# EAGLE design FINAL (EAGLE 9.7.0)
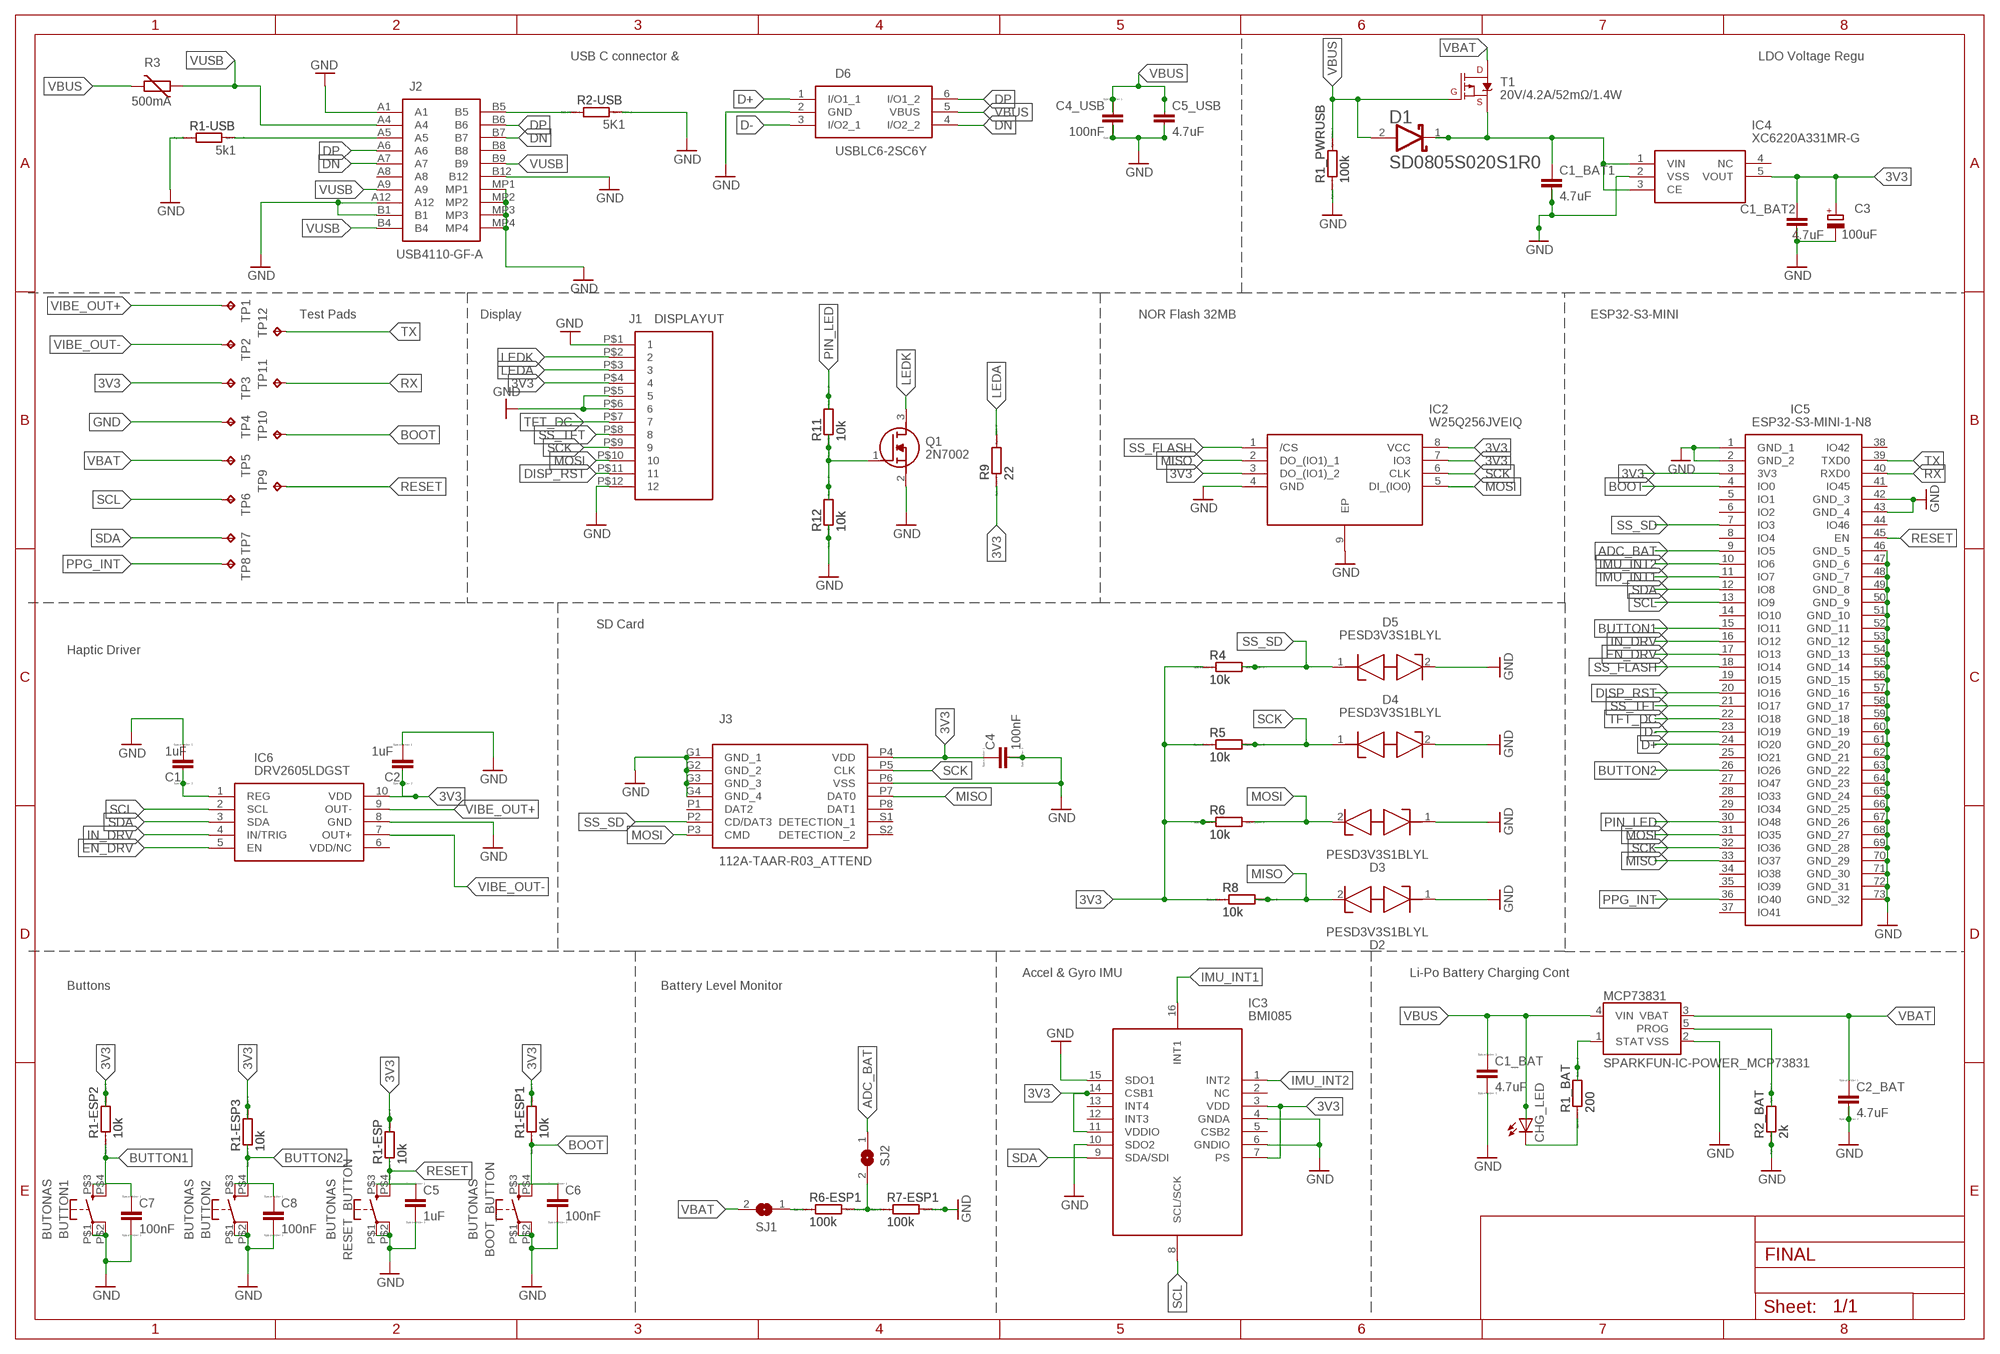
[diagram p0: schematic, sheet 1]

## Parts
BOOT_BUTTON  BUTONAS  [BUTONAS]
BUTTON1  BUTONAS  [BUTONAS]
BUTTON2  BUTONAS  [BUTONAS]
C1  1uF  EAGLE-LTSPICE_CC0402  [EAGLE-LTSPICE_C0402]
C1_BAT  4.7uF  EAGLE-LTSPICE_CC0402  [EAGLE-LTSPICE_C0402]
C1_BAT1  4.7uF  RCL_C-EUC0603  [RCL_C0603]
C1_BAT2  4.7uF  RCL_C-EUC0603  [RCL_C0603]
C2  1uF  EAGLE-LTSPICE_CC0402  [EAGLE-LTSPICE_C0402]
C2_BAT  4.7uF  EAGLE-LTSPICE_CC0402  [EAGLE-LTSPICE_C0402]
C3  100uF  CPOL-EUCT3528  [CT3528]
C4  100nF  EAGLE-LTSPICE_CC0402  [EAGLE-LTSPICE_C0402]
C4_USB  100nF  EAGLE-LTSPICE_CC0402  [EAGLE-LTSPICE_C0402]
C5  1uF  EAGLE-LTSPICE_CC0402  [EAGLE-LTSPICE_C0402]
C5_USB  4.7uF  RCL_C-EUC0603  [RCL_C0603]
C6  100nF  EAGLE-LTSPICE_CC0402  [EAGLE-LTSPICE_C0402]
C7  100nF  EAGLE-LTSPICE_CC0402  [EAGLE-LTSPICE_C0402]
C8  100nF  EAGLE-LTSPICE_CC0402  [EAGLE-LTSPICE_C0402]
CHG_LED  ADAFRUIT_LEDCHIP-LED0603  [ADAFRUIT_CHIP-LED0603]
D1  AVX---SD0805S020S1R0_AVX_SD0805S020S1R0AVX_SD0805S020S1R0_0_0  [AVX---SD0805S020S1R0_AVX_SD0805S020S1R0_0]
D2  PESD3V3S1BLYL  [PESD5V0S1BL315]
D3  PESD3V3S1BLYL  [PESD5V0S1BL315]
D4  PESD3V3S1BLYL  [PESD5V0S1BL315]
D5  PESD3V3S1BLYL  [PESD5V0S1BL315]
D6  USBLC6-2SC6Y  [SOT95P280X145-6N]
IC2  W25Q256JVEIQ  [SON127P800X600X80-9N]
IC3  BMI085  [BMI085]
IC4  XC6220A331MR-G  [SOT95P280X120-5N]
IC5  ESP32-S3-MINI-1-N8  [ESP32S3MINI1N8]
IC6  DRV2605LDGST  [SOP50P490X110-10N]
J1  DISPLAYUT  [DISPLAYUT]
J2  USB4110-GF-A  [USB4110GFA]
J3  112A-TAAR-R03_ATTEND  [112ATAARR03ATTEND]
MCP73831  SPARKFUN-IC-POWER_MCP73831  [SPARKFUN-IC-POWER_SOT23-5]
Q1  2N7002  [SOT96P240X120-3N]
R1-ESP  10k  EAGLE-LTSPICE_RR0402  [EAGLE-LTSPICE_R0402]
R1-ESP1  10k  EAGLE-LTSPICE_RR0402  [EAGLE-LTSPICE_R0402]
R1-ESP2  10k  EAGLE-LTSPICE_RR0402  [EAGLE-LTSPICE_R0402]
R1-ESP3  10k  EAGLE-LTSPICE_RR0402  [EAGLE-LTSPICE_R0402]
R1-USB  5k1  EAGLE-LTSPICE_RR0402  [EAGLE-LTSPICE_R0402]
R1_BAT  200  EAGLE-LTSPICE_RR0402  [EAGLE-LTSPICE_R0402]
R1_PWRUSB  100k  EAGLE-LTSPICE_RR0402  [EAGLE-LTSPICE_R0402]
R2-USB  5K1  EAGLE-LTSPICE_RR0402  [EAGLE-LTSPICE_R0402]
R2_BAT  2k  EAGLE-LTSPICE_RR0402  [EAGLE-LTSPICE_R0402]
R3  500mA  VARISTOR_VARISTORCN1812  [VARISTOR_CT/CN1812]
R4  10k  EAGLE-LTSPICE_RR0402  [EAGLE-LTSPICE_R0402]
R5  10k  EAGLE-LTSPICE_RR0402  [EAGLE-LTSPICE_R0402]
R6  10k  EAGLE-LTSPICE_RR0402  [EAGLE-LTSPICE_R0402]
R6-ESP1  100k  EAGLE-LTSPICE_RR0402  [EAGLE-LTSPICE_R0402]
R7-ESP1  100k  EAGLE-LTSPICE_RR0402  [EAGLE-LTSPICE_R0402]
R8  10k  EAGLE-LTSPICE_RR0402  [EAGLE-LTSPICE_R0402]
R9  22  EAGLE-LTSPICE_RR0402  [EAGLE-LTSPICE_R0402]
R11  10k  EAGLE-LTSPICE_RR0402  [EAGLE-LTSPICE_R0402]
R12  10k  EAGLE-LTSPICE_RR0402  [EAGLE-LTSPICE_R0402]
RESET_BUTTON  BUTONAS  [BUTONAS]
SJ1  SJ  [SJ]
SJ2  SJ  [SJ]
T1  20V/4.2A/52mΩ/1.4W  SPARKFUN-DISCRETESEMI_MOSFET_PCH-SI2309DS  [SPARKFUN-DISCRETESEMI_SOT23-3]
TP1  TPTP20R  [TP20R]
TP2  TPTP20R  [TP20R]
TP3  TPTP20R  [TP20R]
TP4  TPTP20R  [TP20R]
TP5  TPTP20R  [TP20R]
TP6  TPTP20R  [TP20R]
TP7  TPTP20R  [TP20R]
TP8  TPTP20R  [TP20R]
TP9  TPTP20R  [TP20R]
TP10  TPTP20R  [TP20R]
TP11  TPTP20R  [TP20R]
TP12  TPTP20R  [TP20R]

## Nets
3V3 [V_class]: C1_BAT2.1 C2.2 C3.+ C4.1 IC2.3(DO_(IO1)_2) IC2.7(IO3) IC2.8(VCC) IC3.3(VDD) IC3.7(PS) IC3.11(VDDIO) IC3.14(CSB1) IC4.5(VOUT) IC5.3(3V3) IC6.10(VDD) J1.P$4 J3.P4(VDD) R1-ESP1.2 R1-ESP2.2 R1-ESP3.2 R1-ESP.2 R4.1 R5.1 R6.1 R8.1 R9.1 TP3.TP
ADC_BAT: IC5.9(IO5) SJ2.1
BOOT: BOOT_BUTTON.P$3 BOOT_BUTTON.P$4 C6.1 IC5.4(IO0) R1-ESP1.1 TP10.TP
BUTTON1: BUTTON1.P$3 BUTTON1.P$4 C7.1 IC5.15(IO11) R1-ESP2.1
BUTTON2: BUTTON2.P$3 BUTTON2.P$4 C8.1 IC5.26(IO26) R1-ESP3.1
D+: D6.1(I/O1_1) IC5.24(IO20)
D-: D6.3(I/O2_1) IC5.23(IO19)
DISP_RST: IC5.20(IO16) J1.P$11
DN: D6.4(I/O2_2) J2.A7 J2.B7
DP: D6.6(I/O1_2) J2.A6 J2.B6
EN_DRV: IC5.17(IO13) IC6.5(EN)
GND: BOOT_BUTTON.P$1 BOOT_BUTTON.P$2 BUTTON1.P$1 BUTTON1.P$2 BUTTON2.P$1 BUTTON2.P$2 C1.1 C1_BAT1.2 C1_BAT2.2 C1_BAT.2 C2.1 C2_BAT.2 C3.- C4.2 C4_USB.2 C5.2 C5_USB.2 C6.2 C7.2 C8.2 D2.1(K1) D3.1(K1) D4.2(K2) D5.2(K2) D6.2(GND) IC2.4(GND) IC2.9(EP) IC3.4(GNDA) IC3.6(GNDIO) IC3.10(SDO2) IC3.15(SDO1) IC4.2(VSS) IC5.1(GND_1) IC5.2(GND_2) IC5.42(GND_3) IC5.43(GND_4) IC5.46(GND_5) IC5.47(GND_6) IC5.48(GND_7) IC5.49(GND_8) IC5.50(GND_9) IC5.51(GND_10) IC5.52(GND_11) IC5.53(GND_12) IC5.54(GND_13) IC5.55(GND_14) IC5.56(GND_15) IC5.57(GND_16) IC5.58(GND_17) IC5.59(GND_18) IC5.60(GND_19) IC5.61(GND_20) IC5.62(GND_21) IC5.63(GND_22) IC5.64(GND_23) IC5.65(GND_24) IC5.66(GND_25) IC5.67(GND_26) IC5.68(GND_27) IC5.69(GND_28) IC5.70(GND_29) IC5.71(GND_30) IC5.72(GND_31) IC5.73(GND_32) IC6.8(GND) J1.P$1 J1.P$5 J1.P$6 J1.P$12 J2.A1 J2.A12 J2.B1 J2.B12 J2.MP1 J2.MP2 J2.MP3 J2.MP4 J3.G1(GND_1) J3.G2(GND_2) J3.G3(GND_3) J3.G4(GND_4) J3.P6(VSS) MCP73831.2(VSS) Q1.2(S) R1-USB.1 R1_PWRUSB.1 R2-USB.2 R2_BAT.1 R7-ESP1.2 R12.1 RESET_BUTTON.P$1 RESET_BUTTON.P$2 TP4.TP
IMU_INT1: IC3.16(INT1) IC5.11(IO7)
IMU_INT2: IC3.1(INT2) IC5.10(IO6)
IN_DRV: IC5.16(IO12) IC6.4(IN/TRIG)
LEDA: J1.P$3 R9.2
LEDK: J1.P$2 Q1.3(D)
MISO: D2.2(K2) IC2.2(DO_(IO1)_1) IC5.33(IO37) J3.P7(DAT0) R8.2
MOSI: D3.2(K2) IC2.5(DI_(IO0)) IC5.31(IO35) J1.P$10 J3.P3(CMD) R6.2
N$1: J2.A5 R1-USB.2
N$2: J2.B5 R2-USB.1
N$3: C1.2 IC6.1(REG)
N$4: Q1.1(G) R11.1 R12.2
N$6: C1_BAT1.1 D1.1(CATHODE) IC4.1(VIN) IC4.3(CE) T1.2(S)
N$7: R6-ESP1.1 SJ1.1
N$8: R6-ESP1.2 R7-ESP1.1 SJ2.2
N$10: CHG_LED.C R1_BAT.1
N$11: MCP73831.1(STAT) R1_BAT.2
N$15: MCP73831.5(PROG) R2_BAT.2
PIN_LED: IC5.30(IO48) R11.2
PPG_INT: IC5.36(IO40) TP8.TP
RESET: C5.1 IC5.45(EN) R1-ESP.1 RESET_BUTTON.P$3 RESET_BUTTON.P$4 TP9.TP
RX: IC5.40(RXD0) TP11.TP
SCK: D4.1(K1) IC2.6(CLK) IC5.32(IO36) J1.P$9 J3.P5(CLK) R5.2
SCL: IC3.8(SCL/SCK) IC5.13(IO9) IC6.2(SCL) TP6.TP
SDA: IC3.9(SDA/SDI) IC5.12(IO8) IC6.3(SDA) TP7.TP
SS_FLASH: IC2.1(/CS) IC5.18(IO14)
SS_SD: D5.1(K1) IC5.7(IO3) J3.P2(CD/DAT3) R4.2
SS_TFT: IC5.21(IO17) J1.P$8
TFT_DC: IC5.22(IO18) J1.P$7
TX: IC5.39(TXD0) TP12.TP
VBAT [V_class]: C2_BAT.1 MCP73831.3(VBAT) SJ1.2 T1.3(D) TP5.TP
VBUS [V_class]: C1_BAT.1 C4_USB.1 C5_USB.1 CHG_LED.A D1.2(ANODE) D6.5(VBUS) MCP73831.4(VIN) R1_PWRUSB.2 R3.2 T1.1(G)
VIBE_OUT+: IC6.9(OUT-) TP1.TP
VIBE_OUT-: IC6.7(OUT+) TP2.TP
VUSB [V_class]: J2.A4 J2.A9 J2.B4 J2.B9 R3.1
Unconnected: IC3.2(NC) IC3.5(CSB2) IC3.12(INT3) IC3.13(INT4) IC4.4(NC) IC5.5(IO1) IC5.6(IO2) IC5.8(IO4) IC5.14(IO10) IC5.19(IO15) IC5.25(IO21) IC5.27(IO47) IC5.28(IO33) IC5.29(IO34) IC5.34(IO38) IC5.35(IO39) IC5.37(IO41) IC5.38(IO42) IC5.41(IO45) IC5.44(IO46) IC6.6(VDD/NC) J2.A8 J2.B8 J3.P1(DAT2) J3.P8(DAT1) J3.S1(DETECTION_1) J3.S2(DETECTION_2)

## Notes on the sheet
- USB C connector & | LDO Voltage Regu
- Test Pads | Display | NOR Flash 32MB | ESP32-S3-MINI
- SD Card
- Haptic Driver
- Accel & Gyro IMU | Li-Po Battery Charging Cont
- Buttons | Battery Level Monitor

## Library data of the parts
BOOT_BUTTON BUTTON1 BUTTON2 RESET_BUTTON = Library:BUTONAS
C1 C1_BAT C2 C2_BAT C4 C4_USB C5-C8 = Hector_Watch:EAGLE-LTSPICE_C: CAPACITOR, European symbol; SPICEMODEL: NONE; SPICEPREFIX: C
C1_BAT1 C1_BAT2 C5_USB = Hector_Watch:RCL_C-EU: CAPACITOR, European symbol; SPICEPREFIX: C
C3 = Hector_Watch:CPOL-EU: POLARIZED CAPACITOR, European symbol; SPICEPREFIX: C
CHG_LED = Hector_Watch:ADAFRUIT_LED: LED
D1 = Hector_Watch:AVX---SD0805S020S1R0_AVX_SD0805S020S1R0: Schottky Barrier Rectifier Diode; CENTROID_NOT_SPECIFIED: No; DATASHEET: http://datasheets.avx.com/schottky.pdf; DIGIKEY_DESCRIPTION: DIODE SCHOTTKY 20V 1A 0805; DIGIKEY_PART_NUMBER: 478-7800-1-ND; LEAD_FREE: yes; MF: AVX; MOUSER_PART_NUMBER: 581-SD0805S020S1R0; MPN: SD0805S020S1R0; PACKAGE: 0805 (2012 metric); PREFIX: D; ROHS: yes; TEMPERATURE_RANGE_HIGH: +125°C; TEMPERATURE_RANGE_LOW: -55°C
D2-D5 = Hector_Watch:PESD3V3S1BLYL: PESD3V3S1BL - Low capacitance bidirectional ESD protection diode; ARROW_PART_NUMBER: PESD3V3S1BLYL; ARROW_PRICE-STOCK: https://www.arrow.com/en/products/pesd3v3s1blyl/nexperia?region=nac; DESCRIPTION: PESD3V3S1BL - Low capacitance bidirectional ESD protection diode; HEIGHT: 0mm; MANUFACTURER_NAME: Nexperia; MANUFACTURER_PART_NUMBER: PESD3V3S1BLYL; MOUSER_PART_NUMBER: 771-PESD3V3S1BLYL; MOUSER_PRICE-STOCK: https://www.mouser.co.uk/ProductDetail/Nexperia/PESD3V3S1BLYL?qs=vLWxofP3U2zWoKHYJMVoKQ%3D%3D
D6 = Hector_Watch:USBLC6-2SC6Y: Low Cap. ESD Protection Auto SOT-23-6 STMicroelectronics USBLC6-2SC6Y, Dual Uni-Directional TVS Diode Array, 6-Pin SOT-23 Source: Datasheet; ARROW_PART_NUMBER: USBLC6-2SC6Y; ARROW_PRICE-STOCK: https://www.arrow.com/en/products/usblc6-2sc6y/stmicroelectronics?region=nac; DESCRIPTION: Low Cap. ESD Protection Auto SOT-23-6 STMicroelectronics USBLC6-2SC6Y, Dual Uni-Directional TVS Diode Array, 6-Pin SOT-23; HEIGHT: 1.45mm; MANUFACTURER_NAME: STMicroelectronics; MANUFACTURER_PART_NUMBER: USBLC6-2SC6Y; MOUSER_PART_NUMBER: 511-USBLC6-2SC6Y; MOUSER_PRICE-STOCK: https://www.mouser.co.uk/ProductDetail/STMicroelectronics/USBLC6-2SC6Y?qs=gNDSiZmRJS%2FOgDexvXkdow%3D%3D
IC2 = Hector_Watch:W25Q256JVEIQ: 256M-bit Serial Flash Memory with uniform 4KB sectors and Dual/Quad SPI Source: Datasheet; ARROW_PART_NUMBER: W25Q256JVEIQ; ARROW_PRICE-STOCK: https://www.arrow.com/en/products/w25q256jveiq/winbond-electronics?region=nac; DESCRIPTION: 256M-bit Serial Flash Memory with uniform 4KB sectors and Dual/Quad SPI; HEIGHT: 0.8mm; MANUFACTURER_NAME: Winbond; MANUFACTURER_PART_NUMBER: W25Q256JVEIQ; MOUSER_PART_NUMBER: 454-W25Q256JVEIQ; MOUSER_PRICE-STOCK: https://www.mouser.co.uk/ProductDetail/Winbond/W25Q256JVEIQ?qs=qSfuJ%252Bfl%2Fd4o%2FNFUf7yCgA%3D%3D
IC3 = Hector_Watch:BMI085: IMUs - Inertial Measurement Units High-performance IMU BMI085 for virtual and augmented reality applications Source: Datasheet; ARROW_PART_NUMBER: BMI085; ARROW_PRICE-STOCK: https://www.arrow.com/en/products/bmi085/bosch; DESCRIPTION: IMUs - Inertial Measurement Units High-performance IMU BMI085 for virtual and augmented reality applications; HEIGHT: 1mm; MANUFACTURER_NAME: BOSCH; MANUFACTURER_PART_NUMBER: BMI085; MOUSER_PART_NUMBER: 262-BMI085; MOUSER_PRICE-STOCK: https://www.mouser.co.uk/ProductDetail/Bosch-Sensortec/BMI085?qs=y6ZabgHbY%252ByGCM8LfWZyqA%3D%3D
IC4 = Hector_Watch:XC6220A331MR-G: LDO Voltage Regulators Source: Datasheet; DESCRIPTION: LDO Voltage Regulators; HEIGHT: 1.2mm; MANUFACTURER_NAME: Torex; MANUFACTURER_PART_NUMBER: XC6220A331MR-G; MOUSER_PART_NUMBER: 865-XC6220A331MR-G; MOUSER_PRICE-STOCK: https://www.mouser.co.uk/ProductDetail/Torex-Semiconductor/XC6220A331MR-G?qs=AsjdqWjXhJ8ZSWznL1J0gg%3D%3D
IC5 = Hector_Watch:ESP32-S3-MINI-1-N8: WiFi Development Tools - 802.11 [Engineering Samples] SMD Module, ESP32-S3FN8, 8 MB SPI Flash, PCB Antenna Source: Datasheet; DESCRIPTION: WiFi Development Tools - 802.11 [Engineering Samples] SMD Module, ESP32-S3FN8, 8 MB SPI Flash, PCB Antenna; HEIGHT: 2.55mm; MANUFACTURER_NAME: Espressif Systems; MANUFACTURER_PART_NUMBER: ESP32-S3-MINI-1-N8; MOUSER_PART_NUMBER: 356-ESP32-S3-MINI1N8; MOUSER_PRICE-STOCK: https://www.mouser.co.uk/ProductDetail/Espressif-Systems/ESP32-S3-MINI-1-N8?qs=XAiT9M5g4x82rl6F%2FIYUQg%3D%3D
IC6 = Hector_Watch:DRV2605LDGST: ERM & LRA Device Haptic Driver 2-5V BGA9 Texas Instruments DRV2605LDGST Piezo Haptic Motor Driver IC, 5 V, 10-Pin VSSOP Source: Datasheet; ARROW_PART_NUMBER: DRV2605LDGST; ARROW_PRICE-STOCK: https://www.arrow.com/en/products/drv2605ldgst/texas-instruments?region=nac; DESCRIPTION: ERM & LRA Device Haptic Driver 2-5V BGA9 Texas Instruments DRV2605LDGST Piezo Haptic Motor Driver IC, 5 V, 10-Pin VSSOP; HEIGHT: 1.1mm; MANUFACTURER_NAME: Texas Instruments; MANUFACTURER_PART_NUMBER: DRV2605LDGST; MOUSER_PART_NUMBER: 595-DRV2605LDGST; MOUSER_PRICE-STOCK: https://www.mouser.co.uk/ProductDetail/Texas-Instruments/DRV2605LDGST?qs=asCBFxFfL1TjvcNdZsR2BA%3D%3D
J1 = Library:DISPLAYUT
J2 = Hector_Watch:USB4110-GF-A: CONN USB 2.0 TYPE-C R/A SMT Source: Datasheet; DESCRIPTION: CONN USB 2.0 TYPE-C R/A SMT; HEIGHT: 3.26mm; MANUFACTURER_NAME: GCT (GLOBAL CONNECTOR TECHNOLOGY); MANUFACTURER_PART_NUMBER: USB4110-GF-A; MOUSER_PART_NUMBER: 640-USB4110-GF-A; MOUSER_PRICE-STOCK: https://www.mouser.co.uk/ProductDetail/GCT/USB4110-GF-A?qs=KUoIvG%2F9IlYiZvIXQjyJeA%3D%3D
J3 = Hector_Watch:112A-TAAR-R03_ATTEND: Micro SD Card Socket, Push-Push Type, Top Mount, SMT, H=1.83mm, 10u Source: Datasheet; DESCRIPTION: Micro SD Card Socket, Push-Push Type, Top Mount, SMT, H=1.83mm, 10u; HEIGHT: 1.9mm; MANUFACTURER_NAME: ATTEND; MANUFACTURER_PART_NUMBER: 112A-TAAR-R03 ATTEND
MCP73831 = Hector_Watch:SPARKFUN-IC-POWER_MCP73831: MCP73831T Li-Ion, Li-Pol Controller Miniature single cell, fully integrated Li-Ion, Li-polymer charge management controller Datasheet SparkFun Products: SparkFun ESP32 Thing SparkFun 9DoF Razor IMU M0; PROD_ID: IC-09995
Q1 = Hector_Watch:2N7002: N-channel MOSFET,2N7002 0.115A 60V Source: Datasheet; ARROW_PART_NUMBER: 2N7002; ARROW_PRICE-STOCK: https://www.arrow.com/en/products/2n7002/on-semiconductor?region=europe; DESCRIPTION: N-channel MOSFET,2N7002 0.115A 60V; HEIGHT: 1.2mm; MANUFACTURER_NAME: onsemi; MANUFACTURER_PART_NUMBER: 2N7002; MOUSER_PART_NUMBER: 512-2N7002; MOUSER_PRICE-STOCK: https://www.mouser.co.uk/ProductDetail/onsemi-Fairchild/2N7002?qs=0dwsXDNhqlz66WJJhrTFjQ%3D%3D
R1-ESP R1-ESP1-R1-ESP3 R1-USB R1_BAT R1_PWRUSB R2-USB R2_BAT R4-R6 R6-ESP1 R7-ESP1 R8 R9 R11 R12 = Hector_Watch:EAGLE-LTSPICE_R: RESISTOR, European symbol; SPICEMODEL: NONE; SPICEPREFIX: R
R3 = Hector_Watch:VARISTOR_VARISTOR: VARISTOR
SJ1 SJ2 = Hector_Watch:SJ: SMD solder JUMPER
T1 = Hector_Watch:SPARKFUN-DISCRETESEMI_MOSFET_PCH: P-channel MOSFETs Voltage controlled devices that allow control of high current outputs. SparkFun Products: SparkFun ESP32 Thing SparkFun ESP8266 Thing SparkFun Pi Servo HAT V2 DMG2305UX-7 (20V/4.2A/SOT23-3); PROD_ID: TRANS-14715; VALUE: 9A/30V/15mΩ
TP1-TP12 = Hector_Watch:TP: Test pad

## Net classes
0 default: width 0.127 mm
1 V_class: width 0.3 mm

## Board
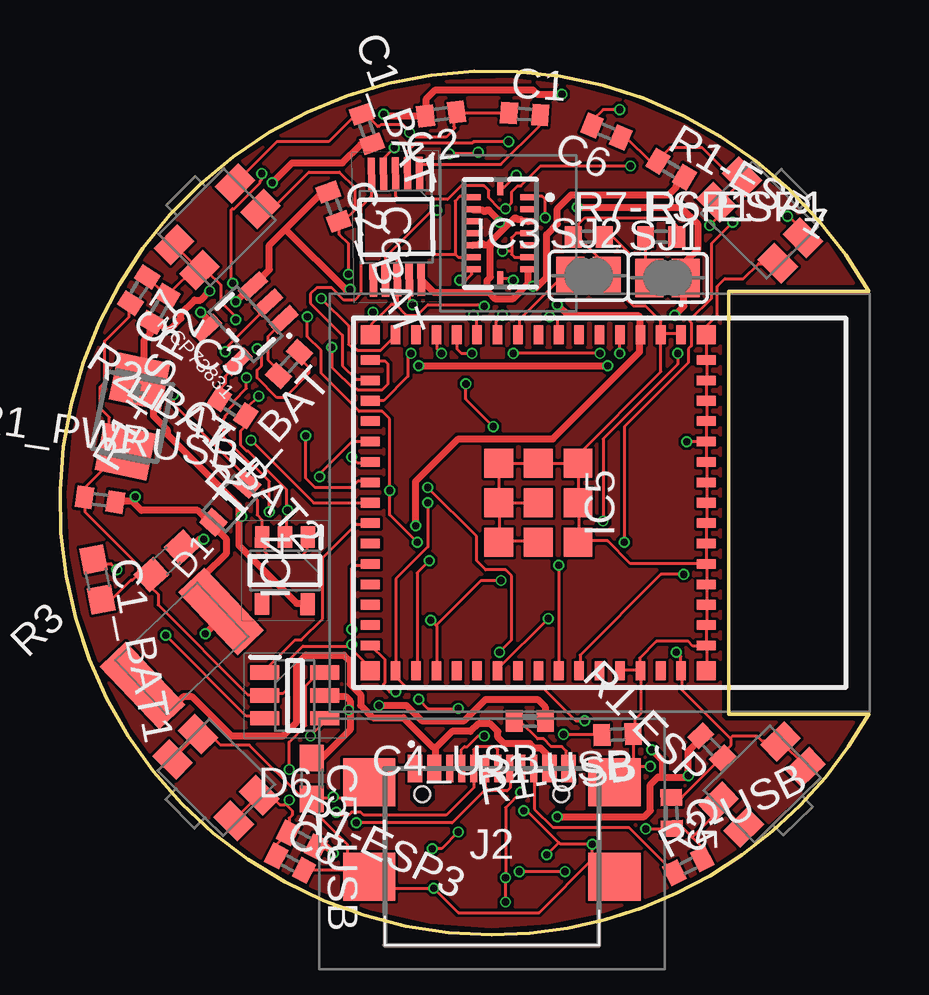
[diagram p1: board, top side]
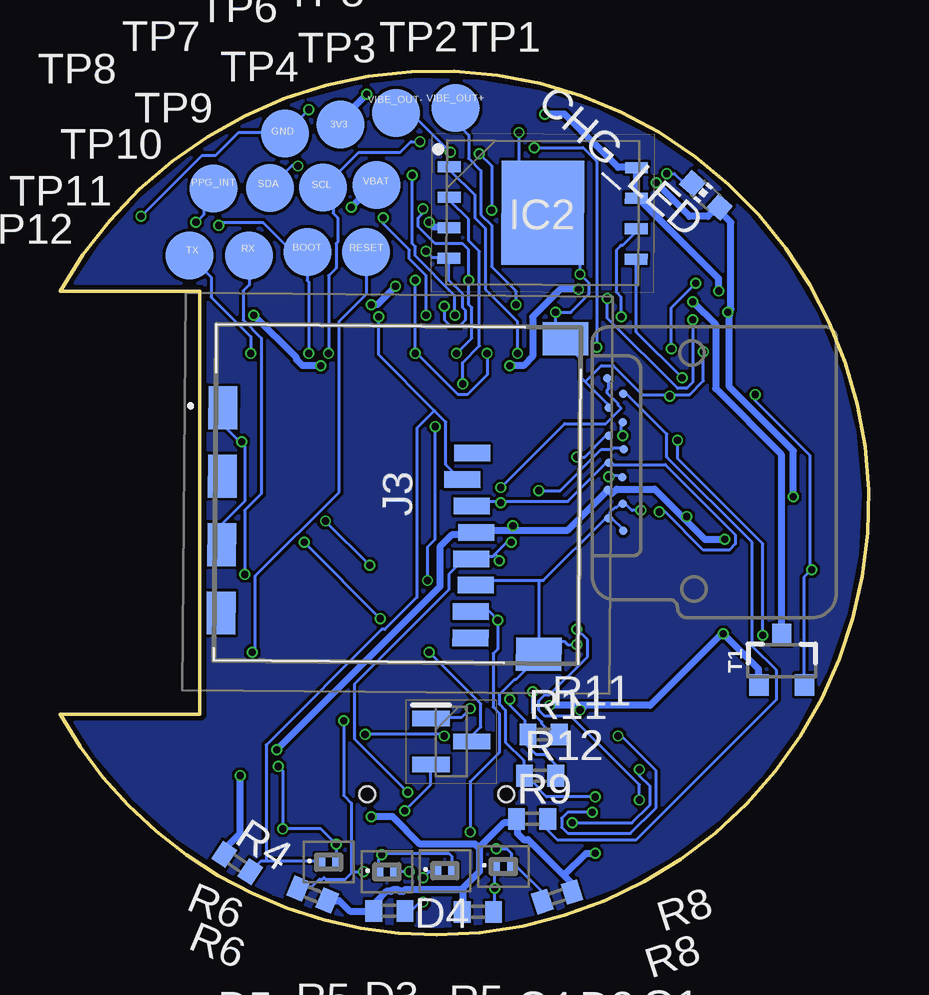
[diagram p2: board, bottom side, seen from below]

Size 33.69 x 35.98 mm. Coordinates in mm from the lower left corner, seen from the top.
Outline: 17.99,0 arc-241 33.69,26.81 27.86,26.81 27.86,9.19 33.69,9.19 arc-61 17.99,0
Copper layers (1*16): Top / Bottom
Stack-up Default Layer Stack: Top User Defined 0.035mm / Dielectric-1 User Defined 1.6mm / Bottom User Defined 0.035mm
Design rules: minimum copper width class=0 5mil, minimum copper width 5mil, minimum drill size 0.3mm, copper clearance wire_polygon to wire_polygon 5mil, copper clearance wire_polygon to pad_smd 5mil, copper clearance wire_polygon to via 5mil, copper clearance pad_smd to pad_smd 5mil, copper clearance pad_smd to via 5mil, copper clearance via to via 5mil, copper clearance smd to pad (same net) 5mil, copper clearance smd to via (same net) 5mil, copper clearance smd to smd (same net) 5mil, dimension clearance 0.2mm, restrict clearance 0mil, via restrict clearance 0mil, drill distance 6mil, keepout clearance 0mil

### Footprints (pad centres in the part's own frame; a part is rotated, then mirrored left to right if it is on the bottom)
BUTONAS = smd 1.4 x 1: P$1 0,0; P$2 0,1.5; P$3 3.6,0; P$4 3.6,1.5
EAGLE-LTSPICE_C0402 = smd 0.7 x 0.9: 1 -0.65,0; 2 0.65,0
RCL_C0603 = smd 1.1 x 1: 1 -0.85,0; 2 0.85,0
CT3528 = smd 2 x 2.2: + -1.5,0; - 1.5,0
ADAFRUIT_CHIP-LED0603 = smd 0.8 x 0.8: A 0,-0.75; C 0,0.75
AVX---SD0805S020S1R0_AVX_SD0805S020S1R0_0 = smd 0.8 x 0.9: 1 -1.05,0; 2 1.05,0
PESD5V0S1BL315 = smd 0.4 x 0.7: 1 -0.35,0; 2 0.35,0
SOT95P280X145-6N = smd 1.2 x 0.6: 1 -1.25,0.95; 2 -1.25,0; 3 -1.25,-0.95; 4 1.25,-0.95; 5 1.25,0; 6 1.25,0.95
SON127P800X600X80-9N = smd 0.95 x 0.45: 1 -3.9,1.905; 2 -3.9,0.635; 3 -3.9,-0.635; 4 -3.9,-1.905; 5 3.9,-1.905; 6 3.9,-0.635; 7 3.9,0.635; 8 3.9,1.905 | smd 3.45 x 4.35: 9 0,0
BMI085 = smd 0.675 x 0.25: 1 1.165,1.5; 2 1.165,1; 3 1.165,0.5; 4 1.165,0; 5 1.165,-0.5; 6 1.165,-1; 7 1.165,-1.5; 9 -1.165,-1.5; 10 -1.165,-1; 11 -1.165,-0.5; 12 -1.165,0; 13 -1.165,0.5; 14 -1.165,1; 15 -1.165,1.5 | smd 0.25 x 0.675: 8 0,-1.915; 16 0,1.915
SOT95P280X120-5N = smd 0.9 x 0.6: 1 -1.4,0.95; 2 -1.4,0; 3 -1.4,-0.95; 4 1.4,-0.95; 5 1.4,0.95
ESP32S3MINI1N8 = smd 0.8 x 0.4: 1 -7,5.95; 2 -7,5.1; 3 -7,4.25; 4 -7,3.4; 5 -7,2.55; 6 -7,1.7; 7 -7,0.85; 8 -7,0; 9 -7,-0.85; 10 -7,-1.7; 11 -7,-2.55; 12 -7,-3.4; 13 -7,-4.25; 14 -7,-5.1; 15 -7,-5.95; 31 7,-5.95; 32 7,-5.1; 33 7,-4.25; 34 7,-3.4; 35 7,-2.55; 36 7,-1.7; 37 7,-0.85; 38 7,0; 39 7,0.85; 40 7,1.7; 41 7,2.55; 42 7,3.4; 43 7,4.25; 44 7,5.1; 45 7,5.95 | smd 0.4 x 0.8: 16 -5.95,-7; 17 -5.1,-7; 18 -4.25,-7; 19 -3.4,-7; 20 -2.55,-7; 21 -1.7,-7; 22 -0.85,-7; 23 0,-7; 24 0.85,-7; 25 1.7,-7; 26 2.55,-7; 27 3.4,-7; 28 4.25,-7; 29 5.1,-7; 30 5.95,-7; 46 5.95,7; 47 5.1,7; 48 4.25,7; 49 3.4,7; 50 2.55,7; 51 1.7,7; 52 0.85,7; 53 0,7; 54 -0.85,7; 55 -1.7,7; 56 -2.55,7; 57 -3.4,7; 58 -4.25,7; 59 -5.1,7; 60 -5.95,7 | smd 1.2 x 1.2: 61 0,0; 66 -1.65,1.65; 67 -1.65,0; 68 -1.65,-1.65; 69 0,-1.65; 70 1.65,-1.65; 71 1.65,0; 72 1.65,1.65; 73 0,1.65 | smd 0.8 x 0.8: 62 -7,7; 63 -7,-7; 64 7,-7; 65 7,7
SOP50P490X110-10N = smd 1.4 x 0.3: 1 -2.2,1; 2 -2.2,0.5; 3 -2.2,0; 4 -2.2,-0.5; 5 -2.2,-1; 6 2.2,-1; 7 2.2,-0.5; 8 2.2,0; 9 2.2,0.5; 10 2.2,1
DISPLAYUT = smd 0.35 x 0.35: P$1 9.059,8.499; P$2 9.717,2.144; P$3 9.053,2.776; P$4 9.707,6.791; P$5 9.072,7.373; P$6 9.654,3.358; P$7 9.066,3.964; P$8 9.652,4.531; P$9 9.039,5.101; P$10 9.66,5.657; P$11 9.095,6.255; P$12 9.674,7.961
USB4110GFA = smd 0.3 x 1.15: A1 -3.35,3.678; A4 -2.55,3.678; A5 -1.25,3.678; A6 -0.25,3.678; A7 0.25,3.678; A8 1.25,3.678; A9 2.55,3.678; A12 3.35,3.678; B1 3.05,3.678; B4 2.25,3.678; B5 1.75,3.678; B6 0.75,3.678; B7 -0.75,3.678; B8 -1.75,3.678; B9 -2.25,3.678; B12 -3.05,3.678 | smd 2.18 x 2: MP1 -5.11,-0.827; MP2 5.11,-0.827; MP3 -5.11,3.103; MP4 5.11,3.103 | hole 0.65: -2.89,2.603; 2.89,2.603
112ATAARR03ATTEND = smd 1.8 x 1.2: G1 10.6,10.4; G2 4.9,10.4; S1 7.75,10.4; S2 2.05,10.4 | smd 1.4 x 1.9: G3 13.6,-3.85; G4 0.45,-2.85 | smd 0.7 x 1.5: P1 8.8,0; P2 7.7,0.4; P3 6.6,0; P4 5.5,-0.2; P5 4.4,0; P6 3.3,-0.2; P7 2.2,0; P8 1.1,0
SPARKFUN-IC-POWER_SOT23-5 = smd 0.55 x 1.2: 1 -0.95,-1.3; 2 0,-1.3; 3 0.95,-1.3; 4 0.95,1.3; 5 -0.95,1.3
SOT96P240X120-3N = smd 1.55 x 0.65: 1 -0.85,0.96; 2 -0.85,-0.96; 3 0.85,0
EAGLE-LTSPICE_R0402 = smd 0.7 x 0.9: 1 -0.65,0; 2 0.65,0
VARISTOR_CT/CN1812 = smd 1.5 x 3.6: 1 -2.25,0; 2 2.25,0
SJ = smd 1.168 x 1.6: 1 -0.762,0; 2 0.762,0
SPARKFUN-DISCRETESEMI_SOT23-3 = smd 0.8 x 0.9: 1 -0.95,-1; 2 0.95,-1; 3 0,1.1
TP20R = smd 2 x 2: TP 0,0

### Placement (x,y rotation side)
BOOT_BUTTON  30.96,29.04 135 top
BUTTON1  7.29,31.3 225 top
BUTTON2  4.69,7.3 315 top
C1  19.36,34.2 356.2 top
C1_BAT  12.79,33.57 109.6 top
C1_BAT1  1.56,14.81 280.9 top
C1_BAT2  4.43,15.58 222.2 top
C2  15.88,34.2 187.3 top
C2_BAT  11.4,30.34 289.8 top
C3  3.02,21.59 258.4 top
C4  16.27,0.96 0 bottom
C4_USB  19.58,8.91 180.4 top
C5  25.48,5.07 271.6 top
C5_USB  10.49,6.51 270.2 top
C6  22.77,33.47 157.6 top
C7  3.28,26.86 237.3 top
C8  9.59,2.98 332.5 top
CHG_LED  6.78,30.81 48.4 bottom
D1  7.1,17.98 228.2 top
D2  15.21,2.85 0 bottom
D3  20.07,2.62 0 bottom
D4  17.65,2.67 0 bottom
D5  22.49,3.03 0 bottom
D6  9.79,9.97 0 top
IC2  13.58,30.08 359.7 bottom
IC3  18.35,29.23 0 top
IC4  9.37,15.17 269.9 top
IC5  19.93,18 270 top
IC6  14.01,29.5 271 top
J1  1.17,25.33 180 bottom
J2  17.99,3.24 0 top
J3  16.59,11.27 89.5 bottom
MCP73831  7.72,25.46 132.5 top
Q1  17.38,8.05 0 bottom
R1-ESP  27.15,7.84 134.4 top
R1-ESP1  25.47,31.9 329 top
R1-ESP2  4.15,26.08 239.7 top
R1-ESP3  10.08,3.95 333.4 top
R1-USB  23.23,8.34 181.8 top
R1_BAT  9.54,23.78 227.9 top
R1_PWRUSB  1.66,18.13 351.4 top
R2-USB  26.18,2.87 26.5 top
R2_BAT  7.19,21.98 146.9 top
R3  5.07,11.93 43.5 top
R4  26.31,2.99 326.1 bottom
R5  19.97,1 0 bottom
R6  23.16,1.68 157.3 bottom
R6-ESP1  25.04,29.08 0 top
R7-ESP1  22.03,29.08 0 top
R8  12.98,1.58 197.8 bottom
R9  14.01,4.83 0 bottom
R11  13.54,8.34 0 bottom
R12  13.69,6.63 0 bottom
RESET_BUTTON  28.49,4.47 44.3 top
SJ1  25.32,27.37 0 top
SJ2  22.03,27.46 0 top
T1  3.61,11.41 0 bottom
TP1  17.21,34.45 0 bottom
TP2  19.68,34.25 0 bottom
TP3  22.01,33.76 0 bottom
TP4  24.31,33.39 0 bottom
TP5  20.51,31.24 0 bottom
TP6  22.73,31.13 0 bottom
TP7  24.95,31.11 0 bottom
TP8  27.29,31.1 0 bottom
TP9  20.94,28.45 0 bottom
TP10  23.38,28.46 0 bottom
TP11  25.81,28.3 0 bottom
TP12  28.3,28.3 0 bottom

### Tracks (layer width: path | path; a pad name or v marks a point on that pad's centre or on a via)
3V3  (via drill 0.3)
  Top 0.3: R1-ESP.2 26.69,8.28 26.69,8.16 26.18,7.65 v26.18,6.63 26.06,6.57 25.1,6.57 | v11.39,3.39 11.13,3.65 10.69,3.65 R1-ESP3.2 | 25.1,6.57 24.91,6.57 24.6,6.25 24.6,5.17 24.34,4.92 v20.72,4.92 | 19.52,27.14 19.52,27.72 IC3.7 | 19.52,27.14 18.88,26.51 18.12,26.51 17.87,26.76 | 17.87,26.76 15.58,26.76 15.07,27.27 IC6.10 | 17.87,28.73 17.67,28.73 17.61,28.8 17.48,28.8 17.42,28.73 17.23,28.73 IC3.11 | 17.87,28.73 17.93,28.67 17.93,27.4 17.8,27.27 17.8,26.89 17.87,26.76 | 18.56,29.49 17.93,28.86 17.87,28.73 | 18.56,29.49 18.95,29.87 19.01,29.87 19.07,29.81 19.2,29.81 19.26,29.75 19.45,29.75 IC3.3 | 18.56,29.49 18.34,29.72 | 18.34,29.72 17.87,30.19 17.8,30.19 17.74,30.13 17.67,30.13 17.61,30.19 17.23,30.19 IC3.14 | v20.72,26.26 21.17,25.81 24.09,25.81 24.15,25.75 24.15,25.05 IC5.3 24.15,24.86 24.15,24.29 20.53,20.67 16.6,20.67 14.82,18.89 v14.82,17.05 | 19.52,27.14 19.64,27.08 v19.71,27.02 19.83,26.95 20.28,27.4 20.28,29.18 20.72,29.62 20.72,30.26 21.29,30.83 25.36,30.83 25.68,31.14 25.68,31.21 25.99,31.52 R1-ESP1.2 | v18.31,29.68 18.34,29.72 | v13.48,34.19 13.55,34.13 15.2,34.13 C2.2 15.26,34.26 15.26,34.83 15.64,35.21 19.71,35.21 19.9,35.02 v20.91,35.02 | v5.99,16.48 5.8,16.48 5.48,16.16 5.1,16.16 C1_BAT2.1 | 7.45,17.43 7.45,17.87 4.47,20.86 4.47,21.05 3.9,21.62 3.9,22.45 3.32,23.02 C3.+ 3.45,23.14 3.51,23.21 3.51,24.8 3.77,25.05 3.77,25.49 R1-ESP2.2 3.96,25.49 4.15,25.49 4.4,25.24 4.59,25.24 5.04,25.68 5.04,25.87 5.61,26.45 5.86,26.45 v6.24,26.83 | 7.45,17.43 7.45,16.22 9.86,13.81 10.31,13.81 IC4.5 | v7.58,17.43 7.45,17.43 | 25.1,6.57 25.1,7.27 v24.66,7.71
  Bottom 0.3: v26.18,6.63 26.18,4.22 26.82,3.59 26.82,3.39 R4.1 | R6.1 22.5,1.43 22.06,1.43 21.61,0.98 20.66,0.98 R5.1 20.53,1.11 20.53,1.36 20.09,1.81 19.9,1.81 19.83,1.87 19.58,1.87 19.52,1.81 19.39,1.81 19.33,1.87 16.91,1.87 | 12.69,2.47 14.18,3.97 14.37,3.97 14.63,4.22 14.63,4.79 R9.1 14.75,4.66 15.2,4.66 16.21,3.65 | 12.69,2.47 12.4,2.19 12.4,1.81 R8.1 | v11.39,3.39 11.77,3.39 12.69,2.47 | 16.91,1.87 16.91,1.93 16.21,2.63 16.21,3.65 | 16.91,1.87 16.91,0.98 C4.1 | v20.72,4.92 19.83,4.92 18.69,3.78 16.41,3.78 16.34,3.71 16.21,3.65 | v20.72,26.26 20.47,26.26 v19.71,27.02 | v18.31,29.68 18.12,29.49 17.48,29.49 IC2.3 | v13.48,34.19 12.66,34.19 10.44,31.97 IC2.8 9.67,31.84 IC2.7 9.55,30.64 6.24,27.34 v6.24,26.83 | v20.91,35.02 21.99,33.94 21.99,33.81 TP3.TP | 14.82,16.86 16.28,16.86 16.34,16.79 J3.P4 16.41,16.67 17.36,16.67 17.87,16.16 17.87,14.51 v24.66,7.71 | 14.82,16.86 12.53,16.86 10.88,18.51 J1.P$4 10.75,18.45 10.69,18.38 10.5,18.57 8.91,18.57 7.67,17.33 | v5.99,16.48 6.82,16.48 7.67,17.33 | v7.58,17.43 7.67,17.33 | v14.82,17.05 14.82,16.86
ADC_BAT
  Top 0.127: IC5.9 19.14,25.05 19.14,25.62 20.91,27.4 21.23,27.4 SJ2.1
BOOT  (via drill 0.3)
  Top 0.127: v23.33,24.22 23.33,24.98 IC5.4 | C6.1 23.39,33.18 23.64,33.18 24.6,32.22 24.85,32.22 R1-ESP1.1 24.91,32.29 25.42,32.8 26.76,32.8 28.28,31.27 | 28.28,31.27 28.41,31.4 28.41,31.52 BOOT_BUTTON.P$3 28.28,31.27 | 28.28,31.27 27.58,30.57 27.39,30.57 BOOT_BUTTON.P$4 27.39,30.51 27.39,29.87 v27.07,29.56
  Bottom 0.127: v23.33,24.22 23.33,27.21 23.39,27.27 23.39,28.41 TP10.TP 23.45,28.41 23.96,28.41 25.23,29.68 26.95,29.68 v27.07,29.56
BUTTON1  (via drill 0.3)
  Top 0.127: C7.1 3.64,27.4 4.34,26.7 4.47,26.7 R1-ESP2.1 4.53,26.7 5.67,27.84 | v10.88,26.51 12.02,25.37 12.02,24.6 12.28,24.35 12.34,24.41 12.4,24.35 13.36,24.35 13.93,24.92 13.93,24.98 IC5.15 | v7.32,25.62 7.32,25.75 6.69,26.38 6.69,27.08 6.12,27.65 5.86,27.65 BUTTON1.P$4 | 5.67,27.84 5.8,27.72 BUTTON1.P$4 | 5.67,27.84 4.78,28.73 BUTTON1.P$3 | 5.67,27.84 BUTTON1.P$4
  Bottom 0.127: v10.88,26.51 10.88,25.68 7.96,22.76 7.58,22.76 7.32,23.02 v7.32,25.62
BUTTON2  (via drill 0.3)
  Top 0.127: C8.1 9.04,3.33 9.04,3.78 9.48,4.22 R1-ESP3.1 9.55,4.28 9.55,4.86 9.67,4.98 9.67,5.17 9.42,5.43 v9.55,5.62 9.36,5.43 9.17,5.43 8.79,5.81 8.34,5.81 BUTTON2.P$4 8.28,5.81 7.26,4.79 BUTTON2.P$3 | v12.15,12.73 12.15,15.27 12.28,15.4 12.91,15.4 IC5.26
  Bottom 0.127: v12.15,12.73 11.71,12.29 11.71,11.59 13.29,10 13.48,10 13.74,9.74 13.74,9.36 13.48,9.11 12.4,9.11 9.55,6.25 v9.55,5.62
D+
  Top 0.127: IC5.24 12.91,17.11 12.34,17.11 10.94,15.71 10.94,13.17 10.05,12.29 9.8,12.29 8.59,11.08 8.59,10.95 D6.1
D-  (via drill 0.3)
  Top 0.127: IC5.23 10.56,18 v7.96,20.6 | v4.4,12.48 7.77,9.11 8.47,9.11 8.53,9.05 D6.3
  Bottom 0.127: v7.96,20.6 7.96,19.84 4.4,16.29 v4.4,12.48
DISP_RST  (via drill 0.3)
  Top 0.127: v10.82,19.08 10.82,19.21 12.15,20.54 12.91,20.54 IC5.20
  Bottom 0.127: v10.82,19.08 10.75,19.08 10.69,19.14 10.44,19.14 10.37,19.08 10.31,19.08 J1.P$11
DN  (via drill 0.3)
  Top 0.127: J2.A7 18.25,6.95 18.25,7.71 18.12,7.84 17.36,7.84 17.23,7.71 17.23,6.95 J2.B7 17.23,6.89 17.23,6.13 16.09,4.98 12.66,4.98 12.53,5.11 12.15,5.11 12.02,4.98 11.64,4.98 v11.52,5.11 | v10.44,8.28 11.01,8.86 11.01,8.98 D6.4
  Bottom 0.127: v10.44,8.28 10.31,8.28 8.85,6.82 8.85,5.3 9.93,4.22 12.53,4.22 12.79,4.47 12.79,4.86 12.53,5.11 v11.52,5.11
DP  (via drill 0.3)
  Top 0.127: 17.77,6.09 17.87,6 18.63,6 18.75,6.13 18.75,6.89 J2.B6 | 17.77,6.09 17.74,6.13 17.74,6.89 J2.A6 | v9.55,6.89 9.55,8.03 10.25,8.73 10.25,10.38 10.75,10.89 11.01,10.89 D6.6 | v12.34,4.66 16.34,4.66 17.77,6.09
  Bottom 0.127: v9.55,6.89 9.55,6.63 9.1,6.19 9.1,5.43 9.86,4.66 v12.34,4.66
EN_DRV
  Top 0.127: IC5.17 12.91,23.14 12.34,23.14 11.77,23.71 11.77,24.98 10.44,26.32 10.44,26.7 10.69,26.95 11.32,26.95 11.83,26.45 12.28,26.45 12.53,26.7 12.53,30.32 12.98,30.76 12.98,31.65 IC6.5
GND  (via drill 0.3)
  Top 0.127: 12.06,12 12.02,12.03 10.12,12.03 9.48,11.4 9.48,10.25 9.29,10.06 8.66,10.06 8.59,10 D6.2 8.53,10 7.83,10 4.09,13.75 4.09,14.19 3.77,14.51 3.77,14.89 C1_BAT2.2 | 12.06,12 12.91,11.14 12.91,11.02 IC5.64 | 3.26,14.95 3.77,14.95 C1_BAT2.2 | 3.26,14.95 3.2,14.95 3.01,14.76 2.94,14.76 2.18,14 1.74,14 C1_BAT1.2 | C7.2 2.88,26.26 2.88,25.75 1.86,24.73 1.86,23.02 1.67,22.83 1.67,21.94 2.05,21.56 2.05,20.48 2.44,20.09 C3.- 2.69,20.09 2.5,20.09 1.04,18.64 1.04,18.25 R1_PWRUSB.1 1.04,18.19 1.04,17.62 3.26,15.4 3.26,14.95 | 3.26,14.95 C1_BAT2.2 | 14.6,33.46 14.82,33.24 16.09,33.24 16.47,33.62 16.41,33.68 16.41,34.19 16.47,34.26 C2.1 16.53,34.26 18.69,34.26 C1.1 | 14.6,33.46 14.31,33.75 13.36,33.75 13.29,33.68 13.23,33.68 12.79,34.13 12.6,34.13 C1_BAT.2 12.53,34.13 12.28,34.13 11.2,33.05 9.04,33.05 7.32,31.34 BUTTON1.P$1 | BUTTON1.P$2 8.4,30.26 8.85,30.26 10.37,31.78 11.64,31.78 12.28,31.14 12.28,30.19 11.83,29.75 11.64,29.75 C2_BAT.2 11.64,29.68 11.64,29.18 12.02,28.8 v12.02,27.52 | 18.82,28.48 18.82,29.05 19.01,29.24 19.45,29.24 IC3.4 | 18.82,28.48 18.82,28.35 18.95,28.22 19.45,28.22 IC3.6 | 18.82,28.48 v18.44,28.48 | 16.47,28.35 16.6,28.22 17.17,28.22 IC3.10 | 16.47,28.35 16.47,30.57 16.66,30.76 17.17,30.76 IC3.15 | 13.26,25.71 13.8,26.26 13.93,26.26 13.96,26.29 | 13.26,25.71 12.98,25.43 12.98,25.05 IC5.63 | 13.96,26.29 14.06,26.38 14.06,27.27 IC6.8 14.06,27.34 14.06,28.22 14.18,28.35 16.47,28.35 | v17.67,26.19 17.48,26.19 17.42,26.26 15.33,26.26 14.88,25.81 14.44,25.81 13.96,26.29 | 9.42,17.68 9.42,18.57 7.83,20.16 7.77,20.16 7.52,20.41 7.52,20.98 7.71,21.18 7.71,21.62 R2_BAT.1 7.77,21.68 7.77,21.94 v8.28,22.45
  Top 0.127: 9.42,17.68 9.42,16.6 IC4.2 | v6.88,24.29 6.88,24.41 8.66,26.19 8.66,26.32 MCP73831.2 | v13.04,25.94 13.26,25.71 | v14.56,33.43 14.6,33.46 | 9.42,17.68 v9.48,17.68 | v12.15,12.09 12.06,12 | 26.34,4.06 26.76,3.65 26.76,3.2 R2-USB.2 | 26.34,4.06 25.99,4.41 25.55,4.41 C5.2 25.49,4.41 v24.41,4.41 | RESET_BUTTON.P$1 28.47,4.47 27.45,5.49 RESET_BUTTON.P$2 27.58,5.3 26.34,4.06 | v19.33,5.17 19.45,5.17 20.79,3.84 | 20.79,3.84 20.85,3.78 v22.18,3.78 22.18,3.33 23.07,2.44 J2.MP2 22.25,3.2 19.96,0.92 16.6,0.92 v15.58,1.93 13.36,1.93 12.91,2.38 J2.MP1 | 20.79,3.84 v20.28,3.33 | 11.96,2.7 12.6,2.7 12.85,2.44 J2.MP1 | 11.96,2.7 10.18,2.7 C8.2 | BUTTON2.P$1 4.72,7.33 5.74,8.35 BUTTON2.P$2 5.8,8.35 6.24,8.35 6.69,7.9 7.9,7.9 10.12,5.68 10.44,5.68 C5_USB.2 | J2.B12 14.88,6.95 14.69,6.95 J2.A1 14.63,6.95 13.48,6.95 12.91,6.38 J2.MP3 12.85,6.32 12.21,5.68 11.39,5.68 | 11.39,5.68 10.75,5.68 | 10.75,5.68 10.5,5.68 C5_USB.2 | 11.96,2.7 11.96,3.78 10.75,4.98 10.75,5.68 | 11.96,2.7 J2.MP1 | 10.75,5.68 C5_USB.2 | IC5.2 25.04,25.05 25.87,25.05 IC5.1 | R7-ESP1.2 22.69,29.05 23.07,29.05 23.71,28.41 23.71,26.51 23.64,26.45 23.9,26.19 24.41,26.19 25.04,25.56 25.04,25.11 IC5.2 | 21.61,18 21.61,16.41 IC5.72 21.68,16.41 22.82,16.41 23.77,15.46 26.88,15.46 IC5.50 | 21.61,18 21.61,19.59 IC5.66 | 21.61,18 IC5.73 | 18.31,18 18.31,16.41 IC5.70 18.37,16.41 19.9,16.41 IC5.71 | 18.31,18 IC5.61 | 18.31,18 18.31,19.59 IC5.68 18.31,19.65 19.9,19.65 IC5.67 19.96,19.65 21.55,19.65 IC5.66 | 18.31,18 IC5.69 | IC5.2 25.04,24.98 25.04,23.46 21.55,19.97 21.55,19.71 IC5.66 | C4_USB.2 18.95,8.86 19.2,8.86 19.9,8.16 20.15,8.16 20.47,7.84 20.91,7.84 21.1,7.65 21.1,6.95 J2.B1 21.17,6.95 21.29,6.95 J2.A12 21.36,6.95 22.5,6.95 23.07,6.38 J2.MP4
  Top 0.127: IC5.42 23.39,11.02 24.15,11.02 IC5.43 | J2.MP4 23.14,6.38 23.9,7.14 23.9,8.35 R1-USB.1 23.96,8.35 23.96,8.98 24.22,9.24 24.22,10.95 IC5.43 | IC5.65 26.95,11.02 26.95,12.03 IC5.46 | IC5.46 26.95,12.09 26.95,12.86 IC5.47 26.95,12.92 26.95,13.75 IC5.48 26.95,13.81 26.95,14.57 IC5.49 26.95,14.63 26.95,15.4 IC5.50 | 26.95,18 26.95,17.17 IC5.52 26.95,17.11 26.95,16.35 IC5.51 26.95,16.29 26.95,15.46 IC5.50 | v23.33,34.38 22.63,34.38 22.18,33.94 22.18,33.75 C6.2 | IC5.56 26.95,20.54 26.95,19.71 IC5.55 26.95,19.65 26.95,18.89 IC5.54 26.95,18.83 26.95,18 | IC5.56 26.95,20.6 26.95,21.37 IC5.57 26.95,21.43 26.95,22.19 IC5.58 26.95,22.25 26.95,23.08 IC5.59 26.95,23.14 26.95,23.91 IC5.60 26.95,23.97 26.95,24.98 IC5.62 26.95,25.05 26.95,25.37 27.39,25.81 27.39,27.02 27.71,27.34 28.47,27.34 29.11,27.97 29.87,27.97 BOOT_BUTTON.P$2 29.93,28.03 30.12,28.03 30.95,28.86 30.95,28.99 BOOT_BUTTON.P$1 30.95,29.05 30.95,29.37 30.38,29.94 v30.31,29.94 | 26.95,18 IC5.53 | v26.12,20.54 26.88,20.54 IC5.56 | IC5.43 24.15,11.08 24.15,11.52 24.85,12.22 26.18,12.22 26.37,12.03 26.88,12.03 IC5.46 | v24.6,7.01 23.83,7.01 J2.MP4 | 11.39,5.68 v11.39,5.74
  Bottom 0.127: J3.G4 13.8,11.65 13.8,11.52 14.69,10.63 14.75,10.63 15.39,10 15.39,9.62 15.14,9.36 15.14,8.03 14.37,7.27 14.37,6.63 R12.1 14.31,6.57 14.18,6.57 13.74,6.13 13.74,6.06 13.42,5.74 v11.39,5.74 | J1.P$1 10.25,16.86 10.25,16.92 10.69,17.36 10.82,17.36 J1.P$12 | J1.P$12 10.88,17.36 10.88,17.43 10.75,17.55 10.75,17.62 10.56,17.81 10.5,17.81 10.37,17.94 10.25,17.94 J1.P$5 10.18,17.94 10.12,17.94 9.86,17.68 v9.48,17.68 | 13.74,14.76 16.15,14.76 16.34,14.57 J3.P6 | 13.74,14.76 13.55,14.76 10.94,17.36 J1.P$12 | 13.74,14.76 13.74,12.22 | 13.74,12.22 13.74,11.71 J3.G4 | v18.44,28.48 18.18,28.22 17.55,28.22 IC2.4 17.48,28.16 17.48,27.27 16.91,26.7 16.91,26.13 16.79,26 16.79,25.62 17.04,25.37 17.42,25.37 17.67,25.62 v17.67,26.19 | 11.8,23.05 11.96,23.21 11.96,23.97 12.6,24.6 12.6,24.8 J3.G3 12.66,24.86 13.04,25.24 v13.04,25.94 12.4,25.94 11.64,26.7 11.64,27.14 v12.02,27.52 12.02,28.54 13.55,30.06 IC2.9 13.61,30.13 14.56,31.08 v14.56,33.43 | 11.8,23.05 10.88,22.13 10.88,22 J1.P$6 | v6.88,24.29 6.88,23.08 7.45,22.51 8.28,22.51 | 8.28,22.51 9.42,22.51 10.63,23.71 11.13,23.71 11.8,23.05 | 8.28,22.51 v8.28,22.45 | v12.15,12.09 12.53,12.09 12.66,12.22 13.74,12.22 | 13.74,12.22 J3.G4 | 20.25,3.3 20.41,3.14 20.41,2.63 D3.1 | 20.25,3.3 20.15,3.39 17.48,3.39 17.36,3.27 17.36,2.7 D4.2 | D5.2 22.18,3.08 v22.18,3.78 22.82,4.41 v24.41,4.41 24.41,6.82 v24.6,7.01 | v19.33,5.17 18.25,6.25 18.25,7.08 Q1.2 | v20.28,3.33 20.25,3.3 | D2.1 15.58,2.82 v15.58,1.93 15.58,0.98 C4.2 | 26.15,20.51 26.88,21.24 26.88,21.94 J3.G1 | 26.15,20.51 25.99,20.35 25.99,18.06 26.95,17.11 26.95,16.29 J3.G2
  Bottom 0.127: v23.33,34.38 24.28,33.43 TP4.TP 24.34,33.43 26.25,33.43 27.2,32.48 27.77,32.48 v30.31,29.94 | v26.12,20.54 26.15,20.51
IMU_INT1  (via drill 0.3)
  Top 0.127: v19.01,31.65 18.5,31.14 18.37,31.14 IC3.16 | v17.23,25.81 17.36,25.68 17.36,25.05 IC5.11
  Bottom 0.127: v19.01,31.65 19.01,28.8 18.88,28.67 18.88,28.29 17.23,26.64 v17.23,25.81
IMU_INT2  (via drill 0.3)
  Top 0.127: v20.22,29.87 20.22,30.64 20.09,30.76 19.52,30.76 IC3.1 | v18.44,25.81 18.18,25.56 18.18,25.05 IC5.10
  Bottom 0.127: v20.22,29.87 20.22,29.62 19.14,28.54 19.14,28.16 18.44,27.46 v18.44,25.81
IN_DRV  (via drill 0.3)
  Top 0.127: v11.32,24.48 11.32,23.65 12.28,22.7 12.34,22.76 12.4,22.7 13.42,22.7 13.67,22.95 13.67,23.78 13.55,23.91 12.98,23.91 IC5.16 | v13.93,32.8 13.48,32.35 13.48,31.72 IC6.4
  Bottom 0.127: v11.32,24.48 11.32,32.22 11.9,32.8 v13.93,32.8
LEDA
  Bottom 0.127: J1.P$3 10.18,22.51 10.05,22.51 8.4,20.86 8.4,19.91 4.85,16.35 4.85,12.03 3.83,11.02 3.83,9.81 9.67,3.97 12.98,3.97 13.42,4.41 13.42,4.79 R9.2
LEDK  (via drill 0.3)
  Top 0.127: v15.33,18.64 17.36,16.6 17.36,15.59 17.74,15.21 18.56,15.21 18.82,14.95 18.82,12.29 v18.31,11.78
  Bottom 0.127: v15.33,18.64 12.66,21.3 10.94,21.3 10.31,21.94 10.44,22.06 10.44,22.13 10.88,22.57 10.88,22.7 10.82,22.76 10.82,23.02 10.88,23.08 10.88,23.14 J1.P$2 | v18.31,11.78 16.15,9.62 16.15,8.66 16.53,8.28 16.53,8.09 Q1.3
MISO  (via drill 0.3)
  Top 0.127: v15.45,13.11 15.67,12.89 | 15.67,12.89 15.71,12.86 15.71,11.02 IC5.33 | v16.91,22.95 16.91,22.32 v18.06,21.18 | v18.37,14.76 17.55,14.76 15.67,12.89 | v15.52,3.59 15.9,3.59 v16.6,4.28
  Bottom 0.127: R8.2 13.61,1.43 13.61,1.81 14.63,2.82 14.82,2.82 D2.2 14.88,2.89 14.88,3.39 15.07,3.59 v15.52,3.59 | J3.P7 16.53,13.49 15.83,13.49 v15.45,13.11 15.45,11.9 15.64,11.71 15.64,9.49 15.39,9.24 15.39,7.59 16.6,6.38 v16.6,4.28 | v16.91,22.95 16.91,23.84 16.21,24.54 16.21,28.48 16.66,28.92 16.66,29.81 17.42,30.57 17.42,30.7 IC2.2 | v18.06,21.18 18.06,16.48 18.37,16.16 v18.37,14.76
MOSI  (via drill 0.3)
  Top 0.127: v21.04,2.63 v19.14,2.63 | v15.33,18 15.33,16.16 13.99,14.82 13.99,11.02 IC5.31 13.99,10.95 13.99,10.76 14.5,10.25 20.15,10.25 21.49,8.92 v21.87,8.92 | v7.77,23.21 7.77,22.76 7.26,22.25 7.26,22.13 7.01,21.87 7.01,21.75 6.88,21.62 6.88,21.56 6.82,21.49 6.82,20.73 8.02,19.52 8.09,19.52 8.72,18.89 v8.72,17.62
  Bottom 0.127: v19.14,2.63 19.71,2.63 D3.2 | v21.04,2.63 21.49,2.63 21.52,2.6 | 21.52,2.6 21.8,2.32 22.63,2.32 22.69,2.38 22.76,2.32 22.88,2.32 23.2,2 23.64,2 23.71,1.93 R6.2 | 15.33,18.06 16.34,18.06 J3.P3 | 15.33,18.06 12.53,18.06 10.94,19.65 10.88,19.65 J1.P$10 10.82,19.65 10.69,19.65 10.63,19.59 8.47,19.59 5.55,16.67 5.55,16.29 5.8,16.03 6.88,16.03 8.47,17.62 v8.72,17.62 | 15.33,18.06 v15.33,18 | v7.77,23.21 9.67,25.11 9.67,28.1 IC2.5 | v21.87,8.92 21.87,5.81 21.55,5.49 21.55,2.63 21.52,2.6
N$1  (via drill 0.3)
  Top 0.127: v20.98,8.35 22.56,8.35 R1-USB.2 | v17.67,8.28 17.42,8.28 16.98,7.84 16.85,7.84 16.72,7.71 16.72,6.95 J2.A5
  Bottom 0.127: v20.98,8.35 17.74,8.35 v17.67,8.28
N$2
  Top 0.127: R2-USB.1 25.55,2.63 23.71,4.47 20.53,4.47 19.77,5.24 19.77,6.89 J2.B5
N$3
  Top 0.127: C1.2 19.96,34.13 19.96,33.68 18.37,32.1 15.07,32.1 15.01,32.03 15.01,31.72 IC6.1
N$4  (via drill 0.3)
  Top 0.127: v16.6,9.43 15.33,9.43 v14.94,9.81
  Bottom 0.127: R12.2 13.04,7.08 13.48,7.52 13.86,7.52 14.25,7.9 14.25,8.28 R11.1 14.31,8.28 14.31,8.92 14.94,9.55 v14.94,9.81 | v16.6,9.43 16.98,9.05 18.18,9.05 Q1.1
N$5
  pour Bottom: -8.11,36.23 47.81,36.23 47.81,-6.5 -7.53,-6.5 -7.53,-6.38 -8.23,-6.38
  pour Top: -3.59,36.34 43.4,36.34 43.4,36.11 44.45,36.11 44.45,-4.87 -3.13,-4.87 -3.13,-2.32
N$6  (via drill 0.3)
  Top 0.127: IC4.1 10.31,16.54 10.31,16.03 10.05,15.78 8.72,15.78 8.53,15.97 8.53,16.48 8.47,16.54 IC4.3 8.4,16.6 8.4,17.3 8.21,17.49 8.21,18.13 7.83,18.51 7.83,18.7 D1.1 7.77,18.76 7.77,19.08 4.72,22.13 v4.72,22.51 | v2.37,15.21 2.12,15.46 1.55,15.46 1.42,15.59 C1_BAT1.1
  Bottom 0.127: T1.2 2.69,10.44 2.69,14.89 v2.37,15.21 2.44,15.21 2.44,19.97 4.72,22.25 v4.72,22.51
N$7
  Top 0.127: R6-ESP1.1 24.41,29.05 24.41,27.52 24.53,27.4 SJ1.1
N$8
  Top 0.127: 21.49,29.18 21.42,29.11 R7-ESP1.1 21.49,29.18 | 21.49,29.18 21.61,29.3 21.61,29.62 21.87,29.87 25.36,29.87 25.68,29.56 25.68,29.11 R6-ESP1.2 | 21.49,29.18 22.76,27.91 22.76,27.46 SJ2.2
N$10  (via drill 0.3)
  Top 0.127: v8.4,31.72 8.4,31.46 8.34,31.4 8.34,31.34 7.26,30.26 7.2,30.26 7.13,30.19 7.13,27.21 v7.2,27.14 | v8.21,24.41 8.4,24.22 8.4,23.71 8.21,23.52 8.21,23.21 9.04,22.38 9.36,22.38 10.37,23.4 10.37,23.65 9.99,24.03 9.99,24.22 R1_BAT.1
  Bottom 0.127: v8.4,31.72 8.09,31.72 7.71,31.34 7.39,31.34 CHG_LED.C | v7.2,27.14 8.21,26.13 v8.21,24.41
N$11
  Top 0.127: R1_BAT.2 9.1,23.33 9.1,23.52 8.66,23.97 8.66,24.92 9.36,25.62 MCP73831.1
N$15
  Top 0.127: R2_BAT.2 6.69,22.38 6.69,22.76 6.88,22.95 6.88,23.27 7.45,23.84 MCP73831.5
PIN_LED  (via drill 0.3)
  Top 0.127: v13.99,10.13 13.74,10.13 13.48,10.38 13.48,10.44 13.55,10.51 13.55,11.46 12.98,12.03 IC5.30
  Bottom 0.127: v13.99,10.13 13.99,9.24 13.61,8.86 13.61,8.79 13.17,8.35 12.91,8.35 R11.2
PPG_INT  (via drill 0.3)
  Top 0.127: v20.34,13.17 18.25,11.08 18.25,11.02 IC5.36 | v23.52,16.35 23.52,21.18 26.18,23.84 26.18,24.41 26.31,24.54 26.31,25.49 26.25,25.56 26.25,25.62 27.14,26.51 27.14,28.8 v28.03,29.68
  Bottom 0.127: v23.52,16.35 v20.34,13.17 | v28.03,29.68 27.71,30 27.71,30.7 27.33,31.08 TP8.TP
RESET  (via drill 0.3)
  Top 0.127: RESET_BUTTON.P$3 31.07,7.01 30.06,8.03 RESET_BUTTON.P$4 29.99,8.09 29.23,8.09 29.04,8.28 28.03,8.28 27.93,8.19 | 27.93,8.19 27.96,8.16 27.96,7.9 27.64,7.59 27.64,7.4 R1-ESP.1 27.58,7.4 25.93,5.74 25.49,5.74 C5.1 | 27.93,8.19 25.93,10.19 25.93,10.95 IC5.45 25.87,11.02 25.87,11.59 v25.68,11.78
  Bottom 0.127: v25.68,11.78 25.55,11.9 25.55,14.95 22.06,18.45 22.06,25.56 20.91,26.7 20.91,28.41 TP9.TP
RX  (via drill 0.3)
  Top 0.127: v25.99,15.02 25.04,15.02 21.68,11.65 21.68,11.02 IC5.40
  Bottom 0.127: v25.99,15.02 25.99,17.68 25.3,18.38 25.3,24.86 26.06,25.62 26.06,26.83 25.8,27.08 25.8,28.29 TP11.TP
SCK  (via drill 0.3)
  Top 0.127: v18.56,1.36 v18.56,2.38 18.56,5.3 v19.2,5.94 | v14.88,16.35 13.74,17.49 v13.74,18.51 13.74,21.49 13.42,21.81 12.47,21.81 10.88,23.4 10.88,24.35 10.31,24.92 v10.31,25.75 | v15.39,15.59 14.88,15.08 14.88,11.02 IC5.32
  Bottom 0.127: v18.56,2.38 18.31,2.63 18.06,2.63 D4.1 | v18.56,1.36 18.69,1.36 19.01,1.05 19.26,1.05 R5.2 | v13.74,18.51 12.85,18.51 11.13,20.22 10.69,20.22 10.63,20.29 10.25,20.29 J1.P$9 | v14.88,16.35 15.07,16.35 15.55,15.87 | 15.55,15.87 15.64,15.78 16.47,15.78 16.53,15.71 J3.P5 16.6,15.65 16.85,15.65 17.48,15.02 17.48,14.38 21.42,10.44 21.42,8.16 v19.2,5.94 | v15.39,15.59 15.39,15.71 15.55,15.87 | v10.31,25.75 10.31,26.57 10.5,26.76 10.5,28.54 10.31,28.73 10.25,28.73 9.74,29.24 9.74,29.37 IC2.6
SCL  (via drill 0.3)
  Top 0.127: v18.88,27.27 18.82,27.34 18.37,27.34 IC3.8 | v15.9,24.22 15.71,24.41 15.71,24.98 IC5.13 | v18.69,33.05 17.23,33.05 17.17,32.99 14.82,32.99 14.44,32.61 14.44,31.72 IC6.2 | v22.5,24.22 v18.88,24.22
  Bottom 0.127: v18.88,27.27 18.88,24.29 18.85,24.25 | 18.85,24.25 17.1,22.51 16.72,22.51 15.9,23.33 v15.9,24.22 | v18.69,33.05 19.07,33.05 19.52,32.61 21.23,32.61 22.69,31.14 TP6.TP 22.69,31.08 22.31,30.7 22.31,30.06 22.12,29.87 22.12,28.86 22.18,28.8 22.18,27.78 22.5,27.46 v22.5,24.22 | v18.88,24.22 18.85,24.25
SDA  (via drill 0.3)
  Top 0.127: v16.66,27.27 16.91,27.27 17.17,27.52 17.17,27.72 IC3.9 | v17.17,24.22 16.72,24.22 16.53,24.41 16.53,24.98 IC5.12 | IC6.3 13.99,31.65 13.99,30.76 14.12,30.64 16.15,30.64 16.72,31.21 17.67,31.21 17.87,31.02 17.87,30.7 18.31,30.26 v18.56,30.26 18.82,30.51 18.82,30.95 19.07,31.21 19.2,31.21 20.02,32.03 v23.77,32.03
  Bottom 0.127: v17.17,24.22 16.53,24.86 16.53,26.13 16.66,26.26 v16.66,27.27 16.66,28.54 16.91,28.8 18.06,28.8 18.75,29.49 18.75,29.87 18.56,30.06 v18.56,30.26 | v23.77,32.03 24.02,32.03 24.91,31.14 TP7.TP
SS_FLASH  (via drill 0.3)
  Top 0.127: v14.63,24.22 14.5,24.1 14.5,23.27 13.48,22.25 12.98,22.25 IC5.18
  Bottom 0.127: v14.63,24.22 14.63,25.56 15.96,26.89 15.96,29.43 16.41,29.87 16.41,30.83 17.42,31.84 17.42,31.97 IC2.1
SS_SD  (via drill 0.3)
  Top 0.127: v20.41,25.75 20.6,25.75 20.72,25.62 20.72,25.05 IC5.7
  Bottom 0.127: 25.1,3.08 25.3,3.08 25.74,2.63 R4.2 | 25.1,3.08 22.88,3.08 D5.1 | v20.41,25.75 20.41,24.16 18.09,21.84 | 18.09,21.84 17.61,21.37 17.61,19.59 16.98,18.95 J3.P2 | 25.1,3.08 25.1,7.9 20.28,12.73 20.15,12.73 18.82,14.06 18.82,21.11 18.09,21.84
SS_TFT  (via drill 0.3)
  Top 0.127: v12.15,19.91 12.4,19.65 12.91,19.65 IC5.21
  Bottom 0.127: v12.15,19.91 11.83,19.91 10.94,20.79 10.88,20.79 J1.P$8
TFT_DC  (via drill 0.3)
  Top 0.127: v10.25,20.79 10.25,19.02 10.63,18.64 12.15,18.64 12.4,18.89 12.91,18.89 IC5.22
  Bottom 0.127: v10.25,20.79 10.31,20.86 10.31,21.18 10.25,21.24 10.25,21.3 J1.P$7
TX  (via drill 0.3)
  Top 0.127: v20.79,15.4 20.79,11.02 IC5.39 | v22.63,17.24 22.63,20.67 25.74,23.78 v25.74,24.22
  Bottom 0.127: v22.63,17.24 v20.79,15.4 | v25.74,24.22 25.74,24.92 27.39,26.57 27.39,27.4 28.28,28.29 TP12.TP
VBAT  (via drill 0.3)
  Top 0.3: v21.55,30.32 25.87,30.32 26.56,29.62 26.56,28.54 26.12,28.1 26.12,27.4 SJ1.2 25.99,27.27 25.99,26.19 v25.61,25.81 | v7.32,26.38 8.02,27.08 MCP73831.3 8.15,27.14 8.72,27.72 8.72,28.73 9.39,29.4 | 9.39,29.4 10.88,30.89 11.13,30.89 C2_BAT.1 | v14.94,23.71 v22.82,23.71 | v12.09,26.89 11.9,26.89 9.39,29.4
  Bottom 0.3: v21.55,30.32 20.66,31.21 20.53,31.21 TP5.TP | v7.32,26.38 6.37,25.43 6.37,22.76 3.64,20.03 3.64,12.54 T1.3 | v25.61,25.81 23.83,24.03 23.83,23.97 23.58,23.71 v22.82,23.71 | v14.94,23.71 14.37,23.71 13.99,24.1 13.99,25.75 12.85,26.89 v12.09,26.89
VBUS  (via drill 0.3)
  Top 0.3: v5.86,25.94 6.24,25.56 6.24,25.37 6.18,25.3 MCP73831.4 | v8.85,31.34 9.67,32.16 11.77,32.16 12.53,32.92 12.98,32.92 C1_BAT.1 | 12.09,9.36 12.09,9.74 11.9,9.94 11.07,9.94 D6.5 | 12.09,9.36 12.09,8.54 10.94,7.4 10.5,7.4 C5_USB.1 | v6.05,12.54 6.69,13.17 6.69,13.43 R3.2 6.69,13.62 6.05,14.25 6.05,15.02 6.94,15.9 6.94,16.48 6.44,16.98 6.44,17.17 D1.2 6.24,17.17 5.74,17.68 3.39,17.68 3.01,18.06 | 3.01,18.06 2.31,18.06 R1_PWRUSB.2 | v13.29,9.55 14.44,9.55 15.07,8.92 16.85,8.92 17.74,9.81 19.9,9.81 20.22,9.49 C4_USB.1 | v12.02,9.36 12.09,9.36 | v3.13,18.25 3.07,18.19 3.01,18.06
  Bottom 0.3: v8.85,31.34 7.45,29.94 6.69,29.94 6.31,30.32 CHG_LED.A 6.18,30.26 6.18,30.13 5.74,29.68 5.74,26.06 v5.86,25.94 5.8,25.81 5.8,22.83 3.13,20.16 v3.13,18.25 | T1.1 4.59,10.44 4.59,11.08 v6.05,12.54 6.18,12.48 9.1,9.55 11.9,9.55 | 11.9,9.55 v13.29,9.55 | v12.02,9.36 11.96,9.36 11.9,9.43 11.9,9.55
VIBE_OUT+  (via drill 0.3)
  Top 0.127: v14.69,26.26 14.56,26.38 14.56,27.27 IC6.9
  Bottom 0.127: v14.69,26.26 14.69,26.83 15.71,27.84 15.71,29.56 16.15,30 16.15,31.84 16.66,32.35 16.66,33.3 17.17,33.81 17.17,34.45 TP1.TP
VIBE_OUT-  (via drill 0.3)
  Top 0.127: v15.71,30.19 15.52,30.19 13.55,28.22 13.55,27.34 IC6.7 | v16.21,32.54 17.36,32.54 v17.42,32.61
  Bottom 0.127: v15.71,30.19 15.71,32.03 v16.21,32.54 | v17.42,32.61 19.01,34.19 19.64,34.19 TP2.TP
VUSB
  Top 0.3: J2.A4 15.45,6.95 15.71,6.95 J2.B9 15.64,7.08 15.64,7.78 | J2.B4 20.28,6.95 20.53,6.95 J2.A9 20.41,7.08 20.41,7.4 20.02,7.78 19.77,7.78 19.58,7.97 18.5,7.97 18.25,8.22 18.25,8.47 17.93,8.79 17.42,8.79 17.1,8.47 16.34,8.47 15.64,7.78 | 15.64,7.78 15.52,7.84 14.31,9.05 13.04,9.05 12.53,9.55 12.53,10 12.09,10.44 12.09,11.4 11.83,11.65 10.25,11.65 9.86,11.27 9.86,8.86 9.29,8.28 7.13,8.28 5.48,9.94 5.17,9.94 4.91,9.68 4.15,9.68 R3.1

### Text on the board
SilkscreenBottom: VIBE_OUT+ | VIBE_OUT- | 3V3 | GND | VBAT | SCL | SDA | PPG_INT | RESET | BOOT | RX | TX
